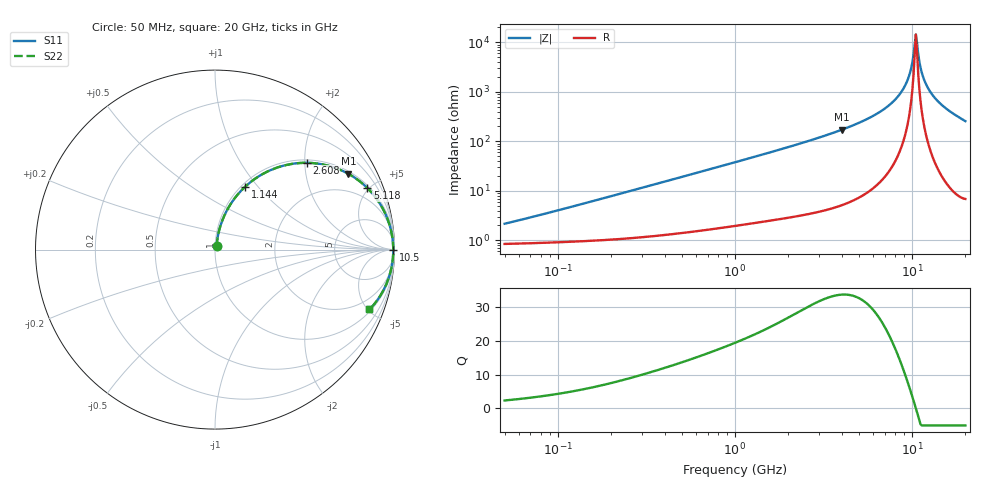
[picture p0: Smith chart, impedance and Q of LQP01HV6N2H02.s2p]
!Murata Part Number: LQP01HV6N2H02
!These Parameters are Measured in Series Mode Connection
!  o--[Z]--o
!Port1  Port2
!  o-------o
!Freq. Start=50[MHz] Stop=20[GHz], 401[Steps]
# Hz S RI R 50
!Freq.(Hz) S11(Real) S11(Imag) S21(Real) S21(Imag) S12(Real) S12(Imag) S22(Real) S22(Imag)
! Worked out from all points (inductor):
!   401 points, 50 MHz to 20 GHz, reference 50 ohm
!   read as one part in series: L = 6.28 nH near 66.46 MHz
!   highest Q = 33.5 at 4.027 GHz (marker M1), where L = 6.83 nH
!   self-resonance near 10.5 GHz
!   S11 on the Smith chart (normalised r, x): 50 MHz: 1.02, +0.04; 1.144 GHz: 1.04, +0.86; 2.608 GHz: 1.07, +2.04; 5.118 GHz: 1.15, +4.90; 10.5 GHz: open; 20 GHz: 1.14, -5.11
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5e7  0.00877 0.0196  0.9912 -0.0196  0.9912 -0.0196  0.00877 0.0196
1.364002e8  0.0122 0.0521  0.9878 -0.0521  0.9878 -0.0521  0.0122 0.0521
3.721004e8  0.0315 0.1363  0.9685 -0.1363  0.9685 -0.1363  0.0315 0.1363
1e9  0.1374 0.3194  0.8626 -0.3194  0.8626 -0.3194  0.1374 0.3194
1.144317e9  0.1693 0.3515  0.8307 -0.3515  0.8307 -0.3515  0.1693 0.3515
2.608132e9  0.5107 0.4835  0.4893 -0.4835  0.4893 -0.4835  0.5107 0.4835
2.728004e9  0.5351 0.4827  0.4649 -0.4827  0.4649 -0.4827  0.5351 0.4827
4.026975e9  0.7428 0.4225  0.2572 -0.4225  0.2572 -0.4225  0.7428 0.4225
5.117541e9  0.8496 0.3423  0.1504 -0.3423  0.1504 -0.3423  0.8496 0.3423
7.442007e9  0.9595 0.1753  0.0405 -0.1753  0.0405 -0.1753  0.9595 0.1753
8.516016e9  0.9804 0.1082  0.0196 -0.1082  0.0196 -0.1082  0.9804 0.1082
9.316812e9  0.9888 0.0623  0.0112 -0.0623  0.0112 -0.0623  0.9888 0.0623
9.745021e9  0.9913 0.0392  0.00865 -0.0392  0.00865 -0.0392  0.9913 0.0392
1.019291e10  0.9928 0.016  0.0072 -0.016  0.0072 -0.016  0.9928 0.016
1.050288e10  0.9931 0.000429  0.00686 -0.000429  0.00686 -0.000429  0.9931 0.000429
1.082228e10  0.993 -0.0152  0.00701 0.0152  0.00701 0.0152  0.993 -0.0152
1.115139e10  0.9923 -0.0308  0.00766 0.0308  0.00766 0.0308  0.9923 -0.0308
1.149051e10  0.9912 -0.0464  0.00882 0.0464  0.00882 0.0464  0.9912 -0.0464
1.201863e10  0.9885 -0.0699  0.0115 0.0699  0.0115 0.0699  0.9885 -0.0699
1.276073e10  0.9831 -0.1012  0.0169 0.1012  0.0169 0.1012  0.9831 -0.1012
1.527346e10  0.9535 -0.1948  0.0465 0.1948  0.0465 0.1948  0.9535 -0.1948
2e10  0.8608 -0.3331  0.1392 0.3331  0.1392 0.3331  0.8608 -0.3331
